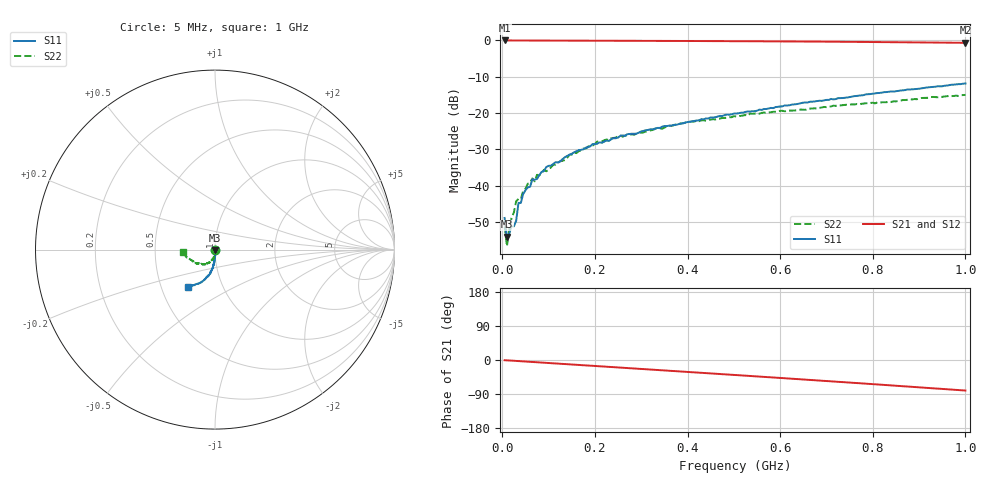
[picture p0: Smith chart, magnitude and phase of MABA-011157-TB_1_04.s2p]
!Agilent Technologies,E5071C,MY46110647,A.11.31
!Date: Thu May 18 15:53:36 2023 DD
!Data & Calibration Information:
!MABA-011157 soldered onto PT-003991 with F connectors, Calibration PCB PT-0003653. Por1 (pin4) Port2 (pin3)
!Freq	S11:SOLT2(ON)	S21:SOLT2(ON)	S12:SOLT2(ON)	S22:SOLT2(ON)
!PortZ  Port1:75+j0  Port2:75+j0
!Above PortZ is port z conversion or system Z0 setting when saving the data.
!When reading, reference impedance value at option line is always used.
# Hz S MA R 75
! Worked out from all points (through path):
!   200 points, 5 MHz to 1 GHz, reference 75 ohm
!   highest |S21| = 0.01 dB at 5 MHz (marker M1); lowest = -0.6 dB at 1 GHz (marker M2)
!   group delay of S21, straight-line fit = 222 ps
!   lowest |S11| = -54.0 dB at 10 MHz (marker M3), VSWR 1.00, Z = 74.8 - j0.251 ohm
!   |S11| at or under -10 dB: start of sweep to end of sweep
!   |S22| runs from -56.6 to -15.0 dB; largest |S21 - S12| = 0.0075
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5000000  0.003607 -92.4  1.001 -0.6  1.002 -0.4  0.002754 -167.1
1e7  0.001986 -122.4  1 -0.9  1 -0.8  0.001476 -139.1
2e7  0.002765 -89.8  0.9994 -1.7  0.9996 -1.7  0.003596 -104.6
2.5e7  0.00276 -93.1  0.9993 -2.1  0.9995 -2.1  0.0043 -87.5
3e7  0.003303 -82.1  0.999 -2.5  0.9987 -2.5  0.006124 -86.7
3.5e7  0.005815 -78.3  0.9986 -2.9  0.9986 -2.8  0.006624 -91.1
4e7  0.005802 -88.9  0.9982 -3.3  0.9985 -3.2  0.006547 -93.3
4.5e7  0.007669 -85.3  0.998 -3.7  0.9982 -3.6  0.00846 -83.9
5.5e7  0.009483 -86.2  0.9976 -4.5  0.9981 -4.4  0.01064 -81.4
6e7  0.009712 -83.4  0.9978 -4.8  0.9977 -4.8  0.01105 -84.6
6.5e7  0.01225 -87.2  0.9976 -5.2  0.9972 -5.2  0.01263 -83.2
7e7  0.01214 -86.2  0.9971 -5.6  0.9972 -5.6  0.01153 -80.0
7.5e7  0.01245 -83.0  0.9972 -6.0  0.9972 -6.0  0.01416 -87.2
9e7  0.01598 -81.9  0.9965 -7.2  0.9962 -7.2  0.01659 -81.6
9.5e7  0.01811 -82.9  0.996 -7.6  0.996 -7.6  0.01586 -80.3
1.75e8  0.03178 -88.1  0.9939 -13.8  0.9937 -13.8  0.03258 -98.4
2.05e8  0.03797 -91.0  0.9923 -16.2  0.9922 -16.1  0.04059 -96.8
3.4e8  0.06262 -93.3  0.987 -26.7  0.9863 -26.8  0.06226 -107.1
5.05e8  0.09866 -95.9  0.9774 -39.7  0.9761 -39.8  0.08994 -121.6
6.7e8  0.1437 -103.0  0.9656 -53.0  0.9625 -53.1  0.1159 -137.2
8.35e8  0.1973 -112.6  0.9499 -66.6  0.9441 -66.7  0.1433 -155.5
1e9  0.2559 -125.4  0.9283 -80.6  0.9212 -80.5  0.1784 -174.9
